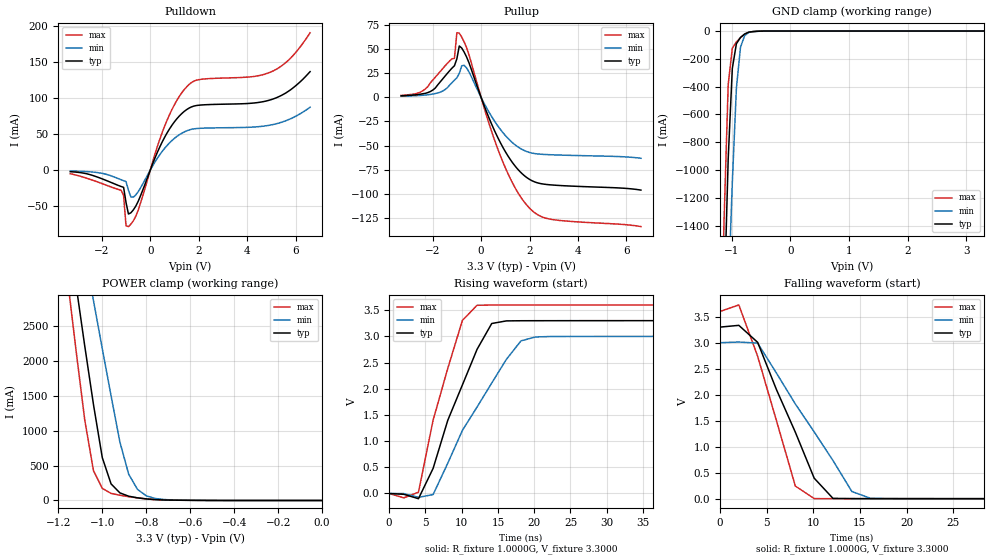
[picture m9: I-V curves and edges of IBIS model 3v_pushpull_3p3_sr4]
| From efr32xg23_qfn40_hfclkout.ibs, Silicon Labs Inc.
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|   Model 3v_pushpull_3p3_sr4
[Model]  3v_pushpull_3p3_sr4
Model_type 3-state
Polarity   Non-Inverting
Enable   Active-High
C_comp   1.6300pF   1.4000pF   2.7000pF
[Temperature Range]   25.0000   0.1250k   -40.0000
[Pullup Reference]   3.3000V   3.0000V   3.6000V
[Pulldown Reference]   0.0V   0.0V   0.0V
[POWER Clamp Reference]   3.3000V   3.0000V   3.6000V
[GND Clamp Reference]   0.0V   0.0V   0.0V
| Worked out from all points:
|   slope of the pulldown table from 0 to 0.495 V, typ, clamps not added: 12.7 ohm
|   slope of the pullup table from 0 to 0.495 V, typ, clamps not added: 15.9 ohm
|   GND clamp passes 1 mA (typ) near -0.52 V on its own axis
|   POWER clamp passes 1 mA (typ) near -0.53 V on its own axis
|   rising waveform, R_fixture 1.0000G, V_fixture 3.3000: 20-80 % time 5.33ns typ, 7.29ns min, 4.1ns max; typ from 0 V to 3.3 V
|   falling waveform, R_fixture 1.0000G, V_fixture 3.3000: 20-80 % time 4.64ns typ, 6.47ns min, 3.56ns max; typ from 3.3 V to 0 V
[Pulldown]
|Voltage   I(typ)   I(min)   I(max)
-3.3V     -2.107mA   -1.127mA   -4.9mA
-1.2V     -22.64mA   -13.29mA   -27.99mA
-1.1V     -23.81mA   -14.62mA   -34.8mA
-1V       -44.79mA   -15.83mA   -77.16mA
-900mV    -60.74mA   -27.73mA   -78.18mA
-800mV    -59.07mA   -37.06mA   -74.82mA
-600mV    -50.02mA   -34.4mA    -64.06mA
700mV     51.87mA    34.37mA    69.6mA
1.5V      83.85mA    54.41mA    115.3mA
5V        97.8mA     62.75mA    136.3mA
5.8V      111.5mA    71.33mA    155.5mA
6.6V      136.5mA    87.15mA    190.3mA
[Pullup]
|Voltage   I(typ)   I(min)   I(max)
-3.3V     1.555mA    1.122mA    1.973mA
-2.5V     3.262mA    1.977mA    5.46mA
-1.9V     9.363mA    3.866mA    20.58mA
-1.1V     32.72mA    17.85mA    40.37mA
-1V       39.81mA    20.25mA    66.83mA
-900mV    53.2mA     24.71mA    66.53mA
-800mV    51.12mA    32.61mA    62.41mA
-600mV    41.88mA    30.52mA    51.53mA
800mV     -47.12mA   -33.35mA   -60.72mA
2V        -84.98mA   -57.12mA   -114.8mA
2.9V      -90.74mA   -59.5mA    -126.4mA
6.6V      -96.11mA   -63.13mA   -133.9mA
[GND_clamp]
|Voltage   I(typ)   I(min)   I(max)
-3.3V     -36.82A    -34.37A    -38.92A
-1.2V     -3.169A    -3.961A    -2.635A
-1.13V    -1.976A    -2.875A    -1.354A
-1.06V    -919.5mA   -1.925A    -386.3mA
-990mV    -269.8mA   -1.092A    -124.2mA
-920mV    -91.07mA   -411.1mA   -78.21mA
-850mV    -46.3mA    -116.2mA   -47.38mA
-780mV    -21.47mA   -33.46mA   -23mA
-710mV    -8.335mA   -10.37mA   -9.191mA
-430mV    -188uA     -421.9uA   -101.6uA
3.3V      1.131nA    22.57uA    998.8pA
[POWER_clamp]
|Voltage   I(typ)   I(min)   I(max)
-3.28V    55.25A     49.02A     61.14A
-1.16V    4.026A     5.102A     3.218A
-1.12V    3.102A     4.316A     2.168A
-1.08V    2.218A     3.57A      1.158A
-1.04V    1.373A     2.863A     426mA
-1V       614.4mA    2.175A     173.2mA
-960mV    237.7mA    1.5A       101.5mA
-920mV    109.2mA    839mA      74.96mA
-880mV    61.4mA     377.7mA    54.07mA
-840mV    37.94mA    159.6mA    37.09mA
-720mV    7.455mA    13.75mA    7.89mA
0V        1.131nA    10.99nA    1.2nA
[Ramp]
| variable   typ   min   max
dV/dt_r  1.9771/5.4802n   1.7964/7.5786n   2.1575/4.1985n
dV/dt_f  1.9778/4.7649n   1.7971/6.6786n   2.1582/3.6151n
R_load = 10.0000k
[Rising Waveform]
R_fixture= 1.0000G
V_fixture= 3.3000
V_fixture_min= 3.0000
V_fixture_max= 3.6000
|time   V(typ)   V(min)   V(max)
0s        1.269uV    2.631uV    739.8nV
4.04ns    -99.66mV   -74.13mV   24.65mV
6.061ns   479.3mV    -20.65mV   1.401V
8.081ns   1.397V     578.1mV    2.388V
10.1ns    2.073V     1.206V     3.306V
12.12ns   2.752V     1.651V     3.593V
14.14ns   3.245V     2.109V     3.598V
18.18ns   3.298V     2.915V     3.599V
20.2ns    3.299V     2.988V     3.599V
200ns     3.3V       3V         3.6V
[Falling Waveform]
R_fixture= 1.0000G
V_fixture= 3.3000
V_fixture_min= 3.0000
V_fixture_max= 3.6000
|time   V(typ)   V(min)   V(max)
0s        3.3V       3V         3.6V
2.02ns    3.334V     3.013V     3.727V
4.04ns    3.007V     2.991V     2.738V
6.061ns   2.096V     2.413V     1.497V
8.081ns   1.278V     1.822V     242.8mV
10.1ns    394.6mV    1.284V     1.668mV
12.12ns   5.25mV     732.7mV    804.1uV
14.14ns   1.422mV    138.1mV    566.9uV
16.16ns   897.2uV    5.876mV    443.4uV
200ns     1.207uV    2.39uV     539.2nV
